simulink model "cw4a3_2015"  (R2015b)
settings: Solver=FixedStepAuto  SolverMode=SingleTasking  StartTime=0.0  StopTime=100  FixedStep=0.01  RelTol=1e-3
libraries: simulink x1

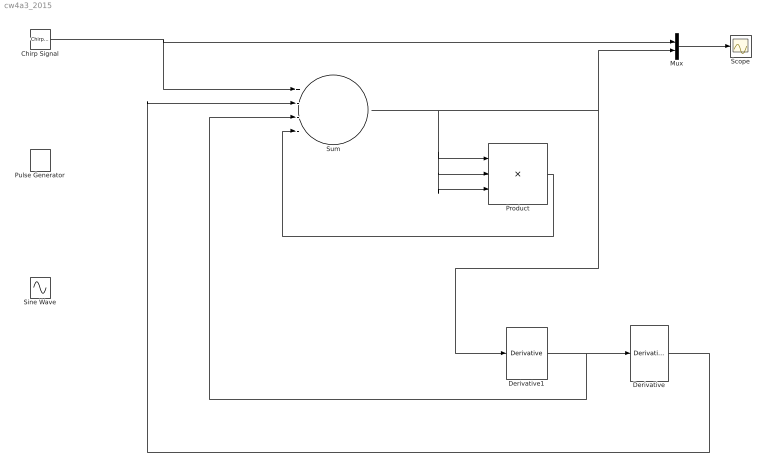
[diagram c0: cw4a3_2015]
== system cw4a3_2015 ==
  Chirp Signal : simulink/Sources/Chirp Signal  f1=0.02  T=100  f2=0.2
  Derivative : Derivative
  Derivative1 : Derivative
  Mux : Mux  Inputs=2
  Product : Product  Inputs=3
  Pulse Generator : DiscretePulseGenerator  PulseType=Time based  Period=10  PulseWidth=50
  Scope : Scope
  Sine Wave : Sin  Frequency=0.11  SampleTime=0
  Sum : Sum  Inputs=+---
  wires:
  Mux/1 -> Scope/1
  Product/1 -> Sum/4
  Sum/1 -> Product/2, Product/3, Product/1, Derivative1/1, Mux/2
  Derivative1/1 -> Sum/3, Derivative/1
  Derivative/1 -> Sum/2
  Chirp Signal/1 -> Mux/1, Sum/1
